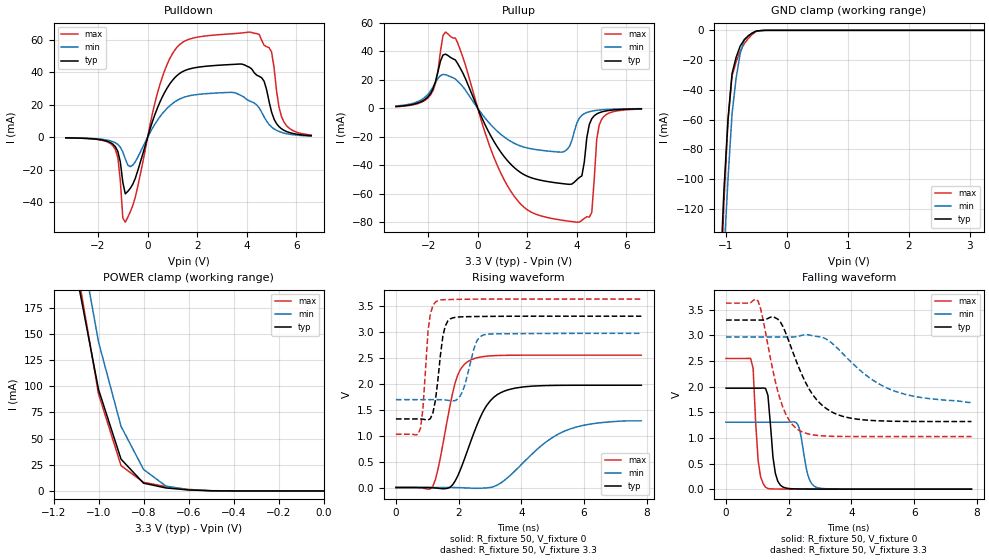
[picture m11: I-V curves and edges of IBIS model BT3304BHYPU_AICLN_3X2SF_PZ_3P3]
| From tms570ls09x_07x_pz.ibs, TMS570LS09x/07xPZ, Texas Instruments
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|   Model Cell BT3304BHYPU_AICLN_3X2SF_PZ_3P3
|BT3304BHYPU_AICLN_3X2SF_PZ_3P3
[Model]   BT3304BHYPU_AICLN_3X2SF_PZ_3P3
Model_type   I/O
Polarity   Non-Inverting
Enable   Active-Low
Vinl =  1.15
Vinh =  1.55
Cref =  15.0001pF
Rref =  101.0000M
Vref =  0V
Vmeas =  1.65
C_comp   1.2p   1.2p   1.2p
[Model Spec]
Vinl   1.15   1.02   1.28
Vinh   1.55   1.45   1.65
[Temperature Range]   25   155   -40
[Voltage Range]   3.3   2.97   3.63
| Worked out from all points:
|   slope of the pulldown table from 0 to 0.495 V, typ, clamps not added: 22.9 ohm
|   slope of the pullup table from 0 to 0.495 V, typ, clamps not added: 26.9 ohm
|   GND clamp passes 1 mA (typ) near -0.53 V on its own axis
|   POWER clamp passes 1 mA (typ) near -0.60 V on its own axis
|   rising waveform, R_fixture 50, V_fixture 0: 20-80 % time 801ps typ, 1.49ns min, 507ps max; typ from 0 V to 1.97 V
|   rising waveform, R_fixture 50, V_fixture 3.3: 20-80 % time 227ps typ, 333ps min, 180ps max; typ from 1.32 V to 3.3 V
|   falling waveform, R_fixture 50, V_fixture 0: 20-80 % time 181ps typ, 234ps min, 147ps max; typ from 1.97 V to 0 V
|   falling waveform, R_fixture 50, V_fixture 3.3: 20-80 % time 941ps typ, 1.62ns min, 605ps max; typ from 3.3 V to 1.32 V
[POWER_clamp]
|   voltage   I(typ)   I(min)   I(max)
-3.3V     3.99A      4.579A     4.788A
-1.1V     209.6mA    262.2mA    219.1mA
-1.067V   172.1mA    222.3mA    177mA
-1.033V   134.5mA    182.3mA    134.9mA
-1V       96.96mA    142.4mA    92.74mA
-900mV    30.4mA     61.8mA     24.2mA
-800mV    7.444mA    20.57mA    8.211mA
-700mV    2.829mA    4.587mA    4.192mA
-600mV    931uA      1.084mA    1.431mA
-500mV    136.9uA    230.8uA    190.6uA
0V        457.7pA    5.751nA    460.2pA
[Pulldown]
|   voltage   I(typ)   I(min)   I(max)
-3.3V     -317.2uA   -283uA     -323.2uA
-1.4V     -4.187mA   -2.645mA   -5.141mA
-1.2V     -8.732mA   -4.393mA   -12.51mA
-1V       -27.63mA   -8.973mA   -49.56mA
-900mV    -34.73mA   -13.26mA   -52.12mA
400mV     18.17mA    10.56mA    27.31mA
1.1V      36.68mA    21.82mA    53.65mA
4.1V      43.08mA    22.4mA     64.63mA
4.7V      34.41mA    12.54mA    56.53mA
5V        15.54mA    6.34mA     52.45mA
5.5V      4.314mA    2.594mA    9.388mA
6.6V      981uA      787.2uA    1.387mA
[Pullup]
|   voltage   I(typ)   I(min)   I(max)
-3.3V     1.246mA    1.609mA    1.076mA
-2V       8.232mA    9.997mA    7.367mA
-1.4V     37.5mA     23.8mA     51.32mA
-900mV    33.96mA    20.66mA    49.39mA
1.4V      -40.56mA   -23.96mA   -60.16mA
3.4V      -52.99mA   -30.87mA   -78.78mA
4V        -50.22mA   -10.35mA   -80.18mA
4.2V      -47.59mA   -4.955mA   -78.93mA
4.6V      -7.373mA   -1.996mA   -73.36mA
4.8V      -3.99mA    -1.436mA   -21.72mA
5V        -2.558mA   -1.08mA    -7.69mA
6.6V      -380.4uA   -267.9uA   -552uA
[GND_clamp]
|   voltage   I(typ)   I(min)   I(max)
-3.3V     -3.259A    -2.879A    -4.965A
-1.1V     -172mA     -209.5mA   -194.3mA
-1.033V   -107.5mA   -151.2mA   -115.6mA
-966.7mV  -59.81mA   -100mA     -61.11mA
-900mV    -29.01mA   -56.02mA   -30.69mA
-833.3mV  -18.19mA   -32.15mA   -21.24mA
-766.7mV  -10.62mA   -15.71mA   -14.04mA
-700mV    -6.305mA   -6.695mA   -9.073mA
-566.7mV  -1.758mA   -1.718mA   -2.644mA
-500mV    -452.5uA   -560.7uA   -673.7uA
-366.7mV  -18.36uA   -44.65uA   -24.3uA
3.233V    436.7pA    2.447uA    352.2pA
[Ramp]
| variable   typ   min   max
dV/dt_f   1.227719/0.9522975n  0.7928572/1.639814n   1.612824/0.6129616n
dV/dt_r   1.196731/0.8085107n  0.7933242/1.548638n   1.549353/0.510054n
R_load = 50
[Rising Waveform]
R_fixture = 50
V_fixture = 0
V_fixture_min = 0
V_fixture_max = 0
|   time   V(typ)   V(min)   V(max)
0s        -1.573uV   -143.3nV   -3.767uV
1.18ns    -5.679mV   -5.52uV    28.37mV
1.336ns   -13.3mV    17.17uV    339mV
1.888ns   125.1mV    -993.2uV   2.013V
2.088ns   391.9mV    -4.273mV   2.302V
2.392ns   896mV      -12.02mV   2.459V
2.896ns   1.581V     -7.185mV   2.53V
3.58ns    1.883V     198.1mV    2.547V
5.392ns   1.969V     1.09V      2.55V
7.828ns   1.97V      1.284V     2.55V
[Rising Waveform]
R_fixture = 50
V_fixture = 3.3
V_fixture_min = 2.97
V_fixture_max = 3.63
|   time   V(typ)   V(min)   V(max)
0s        1.321V     1.693V     1.026V
784ps     1.32V      1.693V     1.143V
864ps     1.316V     1.693V     1.534V
1.024ns   1.298V     1.693V     3.014V
1.18ns    1.439V     1.693V     3.503V
1.336ns   2.056V     1.693V     3.6V
1.572ns   3.108V     1.686V     3.619V
1.808ns   3.267V     1.668V     3.622V
2.796ns   3.295V     2.938V     3.629V
7.828ns   3.3V       2.97V      3.63V
[Falling Waveform]
R_fixture = 50
V_fixture = 0
V_fixture_min = 0
V_fixture_max = 0
|   time   V(typ)   V(min)   V(max)
0s        1.97V      1.307V     2.55V
784ps     1.97V      1.307V     2.552V
864ps     1.97V      1.307V     2.354V
1.024ns   1.97V      1.307V     551.9mV
1.336ns   1.829V     1.307V     12.53mV
1.572ns   310.7mV    1.306V     3.795mV
1.808ns   43.83mV    1.306V     2.504mV
2.292ns   4.682mV    1.255V     968.3uV
2.896ns   1.993mV    32.69mV    224uV
7.828ns   15.71uV    229.2uV    18.31uV
[Falling Waveform]
R_fixture = 50
V_fixture = 3.3
V_fixture_min = 2.97
V_fixture_max = 3.63
|   time   V(typ)   V(min)   V(max)
0s        3.3V       2.97V      3.63V
1.024ns   3.3V       2.97V      3.668V
1.732ns   3.263V     2.97V      1.74V
2.04ns    2.825V     2.969V     1.32V
2.34ns    2.347V     2.99V      1.144V
2.896ns   1.74V      2.98V      1.05V
3.692ns   1.426V     2.664V     1.028V
4.604ns   1.343V     2.159V     1.027V
5.392ns   1.325V     1.91V      1.026V
7.828ns   1.32V      1.692V     1.026V
